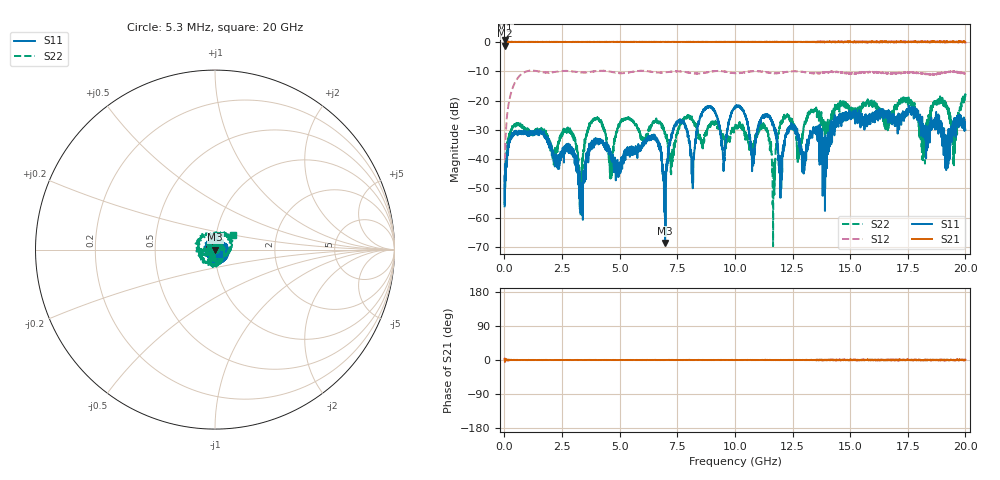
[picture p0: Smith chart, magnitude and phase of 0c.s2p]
!Keysight Technologies,N5232A,MY52221221,A.10.65.11
!Date: Thursday, August 21, 2025 19:54:07
!Correction: S11(Full 2 Port(1,4))
!S41(Full 2 Port(1,4))
!S14(Full 2 Port(1,4))
!S44(Full 2 Port(1,4))
!S2P File: Measurements: S11, S41, S14, S44:
# Hz S  RI  R 50
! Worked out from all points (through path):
!   4000 points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, 5.3 MHz to 20 GHz, reference 50 ohm
!   highest |S21| = 0.51 dB at 30.3 MHz (marker M1); lowest = -1.3 dB at 5.3 MHz (marker M2)
!   lowest |S11| = -68.7 dB at 6.97 GHz (marker M3), VSWR 1.00, Z = 50 - j0.00911 ohm
!   |S11| at or under -10 dB: start of sweep to end of sweep
!   |S22| runs from -69.7 to -17.8 dB; largest |S21 - S12| = 1.3
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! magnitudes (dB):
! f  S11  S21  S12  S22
! 5.3 MHz  -56.1  -1.3  -51.0  -55.2
! 30.3 MHz  -49.8  0.5  -35.9  -46.9
! 645.3 MHz  -30.8  0.0  -11.6  -28.2
! 2.825 GHz  -36.4  0.0  -10.0  -31.0
! 3.34 GHz  -57.7  0.0  -10.4  -44.8
! 3.885 GHz  -34.4  0.0  -10.1  -26.2
! 4.6 GHz  -37.6  0.0  -10.2  -43.3
! 6.67 GHz  -34.1  0.0  -10.5  -27.4
! 6.97 GHz  -68.7  0.0  -10.4  -31.2
! 7.51 GHz  -27.3  0.0  -10.1  -30.2
! 8.16 GHz  -44.6  0.0  -10.7  -26.2
! 8.67 GHz  -23.3  0.0  -10.6  -32.9
! 9.51 GHz  -41.5  0.0  -10.0  -32.1
! 10.01 GHz  -22.4  0.0  -10.7  -28.8
! 10.78 GHz  -39.7  0.0  -10.0  -36.9
! 11.68 GHz  -28.0  0.0  -10.6  -45.8
! 12.06 GHz  -39.1  0.0  -10.4  -27.4
! 13.34 GHz  -30.9  0.0  -10.7  -23.4
! 16.67 GHz  -25.8  0.0  -10.7  -28.4
! 18.93 GHz  -27.6  -0.1  -10.7  -20.6
! 19.54 GHz  -27.1  0.0  -10.3  -37.8
! 20 GHz  -30.0  -0.1  -10.7  -18.2
